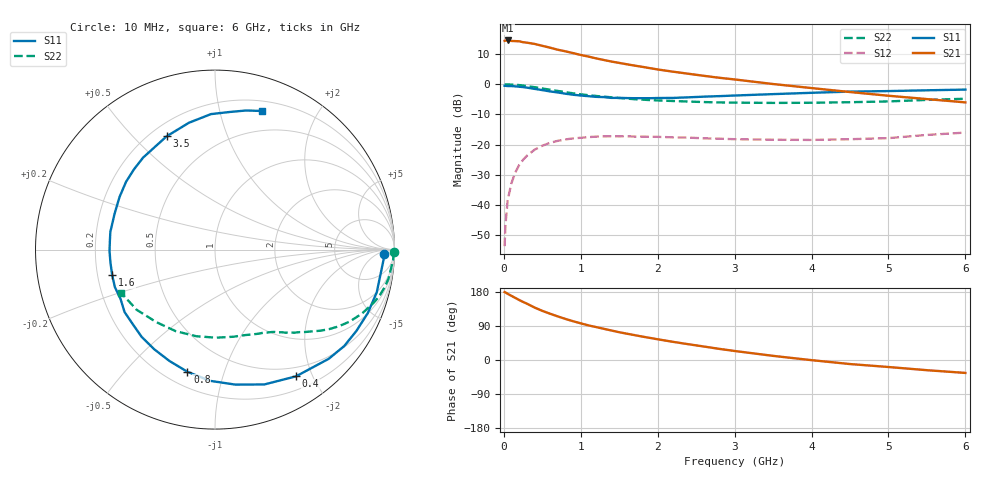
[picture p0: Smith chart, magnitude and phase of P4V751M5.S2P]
! SIEMENS Small Signal Semiconductors
! BFP182
! Si NPN RF Bipolar Junction Transistor in SOT143
! VCE = 0.75 V  IC = 1.5 mA
! Common Emitter S-Parameters:  March  1996
# GHz  S  MA  R  50
!  f  S11  S21  S12  S22
! GHz  MAG  ANG  MAG  ANG  MAG  ANG  MAG  ANG
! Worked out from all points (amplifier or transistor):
!   36 points, 10 MHz to 6 GHz, reference 50 ohm
!   highest |S21| = 14.5 dB at 50 MHz (marker M1)
!   |S21| within 3 dB of that: start of sweep to 691.2 MHz
!   unconditionally stable (mu >= 1): 2.245 GHz to end of sweep
!   at 250 MHz: K = 0.12, MSG = 19.5 dB, |S12| = -25.0 dB
!   at 1.4 GHz: K = 0.64, MSG = 12.3 dB, |S12| = -17.2 dB
!   at 6 GHz: K = 1.18, MAG = 2.4 dB, |S12| = -16.0 dB
!   S11 on the Smith chart (normalised r, x): 10 MHz: 28, -13; 400 MHz: 0.37, -1.77; 800 MHz: 0.29, -0.76; 1.6 GHz: 0.26, -0.11; 3.5 GHz: 0.26, +0.63; 6 GHz: 0.29, +1.35
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0.01  0.9426 -1.5  5.217 179.3  0.0021 85.3  0.9967 -0.7
0.02  0.9416 -3.1  5.253 178.4  0.0045 84.7  0.9945 -1.3
0.05  0.9334 -7.6  5.295 174.6  0.0122 88.1  0.9943 -3.2
0.1  0.9321 -14.8  5.198 169.2  0.0234 80.6  0.9856 -6.5
0.2  0.9089 -29.9  5.131 158.2  0.0464 72.2  0.9671 -12.7
0.3  0.8786 -43.8  4.864 148.7  0.0657 64.0  0.9332 -18.4
0.4  0.8381 -57.4  4.638 138.4  0.0828 56.4  0.8934 -23.5
0.5  0.8 -69.9  4.316 129.7  0.0962 49.3  0.8508 -28.1
0.6  0.7608 -81.4  4.025 122.2  0.1074 43.4  0.8123 -31.7
0.7  0.7316 -92.2  3.723 115.1  0.1158 38.1  0.7748 -34.9
0.8  0.6979 -102.7  3.503 108.4  0.1222 33.3  0.7407 -37.6
0.9  0.6706 -112.2  3.272 102.3  0.1272 29.5  0.7071 -40.1
1.1  0.635 -130.1  2.866 91.3  0.1335 22.5  0.6583 -44.3
1.4  0.5937 -152.4  2.371 77.8  0.1381 14.3  0.6078 -49.6
1.6  0.5902 -166.1  2.137 69.4  0.138 10.4  0.58 -52.7
1.8  0.5876 -179.2  1.939 61.8  0.136 7.7  0.5563 -55.7
2.2  0.5941 160.3  1.612 47.9  0.1324 2.9  0.5281 -62.4
2.8  0.6356 135.2  1.279 29.4  0.1258 -0.4  0.5002 -73.6
3.5  0.6863 113.1  1.008 10.9  0.1209 -0.3  0.4909 -89.3
4.5  0.7553 91.7  0.743 -10.7  0.1233 3.4  0.5043 -115.7
5.5  0.7938 77.5  0.568 -26.9  0.1451 7.3  0.5504 -142.5
6  0.8151 71.4  0.501 -34.1  0.1587 5.5  0.5757 -155.2
